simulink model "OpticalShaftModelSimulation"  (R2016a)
settings: Solver=VariableStepAuto  StartTime=0.0  StopTime=10.0  RelTol=1e-3
libraries: vexarmcortexlib x4

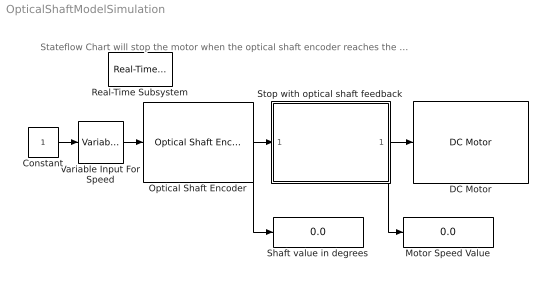
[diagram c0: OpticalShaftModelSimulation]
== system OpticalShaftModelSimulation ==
  note: Stateflow Chart will stop the motor when the optical shaft encoder reaches the set-point
  Constant : Constant
  DC Motor : vexarmcortexlib/DC Motor  motor=7  scaleFactor=1/13.5  SimulationOut=on
  Motor Speed Value : Display
  Optical Shaft Encoder : vexarmcortexlib/Optical Shaft Encoder  topPort=11  bottomPort=12  resetOption=No reset  inputPortSim=on  SampleTime=0.2
  Real-Time Subsystem : vexarmcortexlib/Utilities/Real-Time Subsystem  x=1
  Shaft value in degrees : Display
  Stop with optical shaft feedback : Stateflow chart  TreatAsAtomicUnit=on
  Variable Input For Speed : vexarmcortexlib/Utilities/Variable Input  low=-127  gain=5  high=127
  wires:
  Stop with optical shaft feedback/1(speed) -> Motor Speed Value/1, DC Motor/1
  Optical Shaft Encoder/1 -> Shaft value in degrees/1, Stop with optical shaft feedback/1(shaft)
  Variable Input For Speed/1 -> Optical Shaft Encoder/1
  Constant/1 -> Variable Input For Speed/1

== stateflow chart OpticalShaftModelSimulation/Stop with optical shaft 
feedback ==
  state <!DOCTYPE HTML PUBLIC "-//W3C//DTD HTML 4.0//EN" "http://www.w3.org/TR/REC-html40/strict.dtd"> [group]
    <html><head><meta name="qrichtext" content="1" /><style type="text/css">
    p, li { white-space: pre-wrap; }
    </style></head><body style=" font-family:'Helvetica'; font-size:12px; font-weight:400; font-style:normal;">
    <p style=" margin-top:0px; margin-bottom:0px; margin-left:0px; margin-right:0px; -qt-block-indent:0; text-indent:0px;">Stateflow Chart <span style=" font-style:italic;">transitions</span> to <span style=" font-weight:600;">Stop</span> when</p>
    <p style=" margin-top:0px; margin-bottom:0px; margin-left:0px; margin-right:0px; -qt-block-indent:0; text-indent:0px;">the value of the input variable <span style=" font-style:italic;">shaft</span> </p>
    <p style=" margin-top:0px; margin-bottom:0px; margin-left:0px; margin-right:0px; -qt-block-indent:0; text-indent:0px;">reaches 360 ticks or degrees</p></body></html>
  state Drive_Forward
    during:
    speed = 30;
  state Stop
    during:
    speed =0;
  (default) -> Drive_Forward : {speed = 0;}
  Drive_Forward -> Stop : [shaft > 360]
  data: shaft input; speed output
